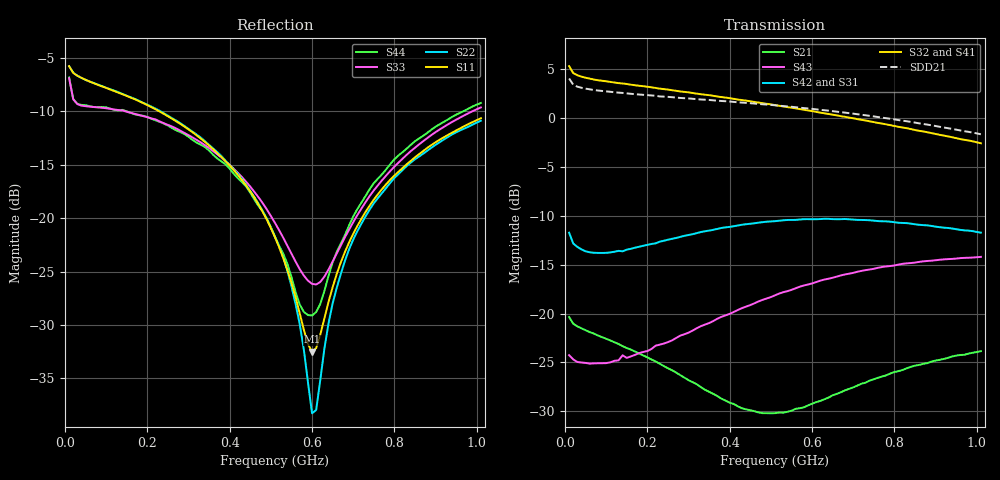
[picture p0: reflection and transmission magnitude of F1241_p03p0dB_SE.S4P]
! Integrated Device Technology
! Corporate Headquarters
! 6024 Silver Creek Valley Road
! San Jose, CA 95138  USA
! Phone:  1-408-284-8200
! Toll Free:  1-800-223-1366
! Webpage:  http://www.idt.com/
! Timing and RF Division
! 515 Groton Road, Suite 102
! Westford, MA 01886-6024
! Device:  F1241
! Description: Dual Intermediate Frequency Digital Variable Gain Amplifier
! Frequency:  10.0 -  500.00 MHz
! Package:  5x5 mm QFN Plastic Package: 32 pin
! Ports:  8 RF, 20 DC
!  Pin  1  = GA3  Pin 17  = RF OUT_B+
!  Pin  2  = GA4  Pin 18  = RF OUT_B-
!  Pin  3  = GA5  Pin 19  = STBY_B
!  Pin  4  = ISET_A  Pin 20  = Ground
!  Pin  5  = ISET_B  Pin 21  = Ground
!  Pin  6  = GB5  Pin 22  = STB_A
!  Pin  7  = GB4  Pin 23  = RF OUT_A-  = Port 4
!  Pin  8  = GB3  Pin 24  = RF OUT_A+  = Port 3
!  Pin  9  = GB2  Pin 25  = NO CONNECT
!  Pin 10  = GB1  Pin 26  = NO CONNECT
!  Pin 11  = RF IN_B+  Pin 27  = VCC
!  Pin 12  = RF IN_B-  Pin 28  = Ground
!  Pin 13  = Ground  Pin 29  = RF IN_A-  = Port 2
!  Pin 14  = VCC  Pin 30  = RF IN_A+  = Port 1
!  Pin 15  = NO CONNECT  Pin 31  = GA1
!  Pin 16  = NO CONNECT  Pin 32  = GA2
! State:  17
! Gain State:  3.0 dB
! Voltages:  Vcc = +5.00 Volts  Icc approximately 160.0 mA or 80 mA per channel.
! Data:  The device was measured on a custom evaluation board which has
!  individual transmission lines to the RF pins.  Data was collected
!  using a calibrated network analyzer.  The evaluation board was
!  de-embedded using a port reference technique.
!  The reference plane is the edge of the package pin.
!  Only Channel A was measured.
!  This data is in single-ended operation.  If your needs are balanced
!  or differential S-parameters then this file needs to be used a
!  linear simulator.
! Misc:  Lot Code  160028MY
!  Action Tracker AT004
! Date Measured:  2014-08-14
! Date:  2014-08-28  MJV
! Note:
!  Integrated Device Technology supplies this data as a sample of measured
!  data at the package pin for this product.  Your particular data for this
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# Hz S dB R 50
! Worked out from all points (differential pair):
!   101 points, 10 MHz to 1.01 GHz, reference 50 ohm
!   strongest paths, dB at 10 MHz, 260 MHz, 510 MHz, 760 MHz, 1.01 GHz:
!     S32: 5.3, 2.8, 1.3, -0.5, -2.6
!     S41: 5.3, 2.8, 1.2, -0.7, -2.8
!     S42: -11.7, -12.4, -10.6, -10.5, -11.7
!     S31: -11.7, -12.3, -10.6, -10.6, -11.9
!     S43: -24.3, -22.7, -18.1, -15.3, -14.2
!     S21: -20.4, -25.8, -30.2, -26.6, -23.9
!   taken as a pair (ports 2,1 in; 3,4 out), SDD21 dB: 4.0, 2.1, 1.3, 0.1, -1.7
!   lowest |S11| = -32.5 dB at 600 MHz (marker M1), VSWR 1.05, Z = 48.3 - j1.54 ohm
!   |S11| at or under -10 dB: 228.7 MHz to end of sweep
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1e7  -5.79 -14.3  -20.35 -18.0  -38.92 2.3  -19.54 12.1
     -20.36 -18.0  -5.78 -14.1  -19.56 11.8  -38.93 2.5
     -11.73 160.3  5.29 172.6  -6.91 -31.2  -24.34 -175.1
     5.33 172.7  -11.74 160.4  -24.26 -175.1  -6.84 -31.1
2.2e8  -9.82 -29.5  -24.92 -27.0  -36.30 28.1  -20.12 -14.5
       -24.90 -27.5  -9.76 -27.5  -20.12 -14.5  -36.29 27.3
       -12.82 89.3  3.07 142.6  -10.77 -21.6  -23.42 138.9
       3.07 142.0  -12.83 89.5  -23.29 138.8  -10.85 -20.3
4.4e8  -16.97 -50.8  -29.56 -12.9  -32.39 24.3  -20.04 -27.9
       -29.81 -13.6  -16.89 -45.3  -19.92 -27.5  -32.40 22.5
       -10.90 35.3  1.77 113.2  -16.61 -46.6  -19.56 105.3
       1.71 112.2  -10.87 34.6  -19.29 104.6  -17.06 -43.5
5.4e8  -24.84 -72.0  -29.63 4.7  -31.14 19.7  -20.03 -35.0
       -30.06 4.9  -24.92 -59.0  -19.83 -34.7  -31.13 17.2
       -10.51 15.5  1.11 100.7  -22.58 -74.9  -17.97 91.0
       1.02 99.6  -10.44 14.5  -17.71 90.2  -24.27 -70.6
6e8  -32.51 -137.6  -28.92 12.5  -30.51 16.3  -20.06 -39.6
     -29.23 13.6  -38.26 -125.0  -19.83 -39.2  -30.46 14.0
     -10.42 4.6  0.69 93.4  -26.15 -122.1  -17.15 82.6
     0.60 92.3  -10.36 3.4  -16.92 81.9  -29.11 -137.4
7.3e8  -19.41 136.3  -26.81 19.4  -29.26 8.5  -20.31 -49.4
       -27.07 21.6  -19.82 132.1  -19.96 -49.2  -29.28 5.1
       -10.55 -16.4  -0.27 78.3  -18.50 159.4  -15.87 65.1
       -0.41 77.2  -10.44 -18.1  -15.56 64.4  -17.92 149.4
1.01e9  -10.65 118.2  -23.95 15.4  -27.53 -11.1  -21.45 -69.1
        -23.85 16.7  -10.89 117.6  -20.83 -69.2  -27.52 -14.7
        -11.88 -51.3  -2.59 49.4  -9.64 130.6  -14.50 32.8
        -2.80 48.4  -11.73 -54.4  -14.21 32.4  -9.23 126.5
